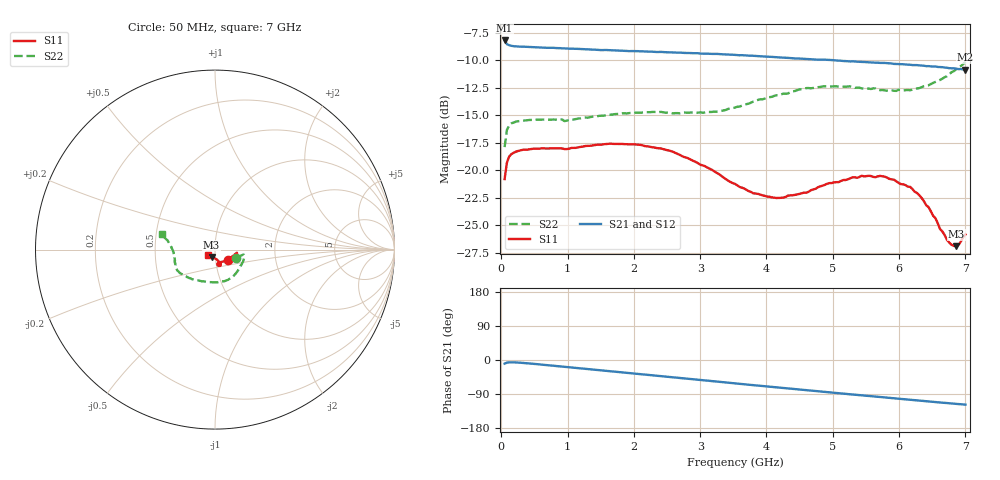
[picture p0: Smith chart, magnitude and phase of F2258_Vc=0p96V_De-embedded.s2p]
! Integrated Device Technology
! Corporate Headquarters
! 6024 Silver Creek Valley Road
! San Jose, CA 95138  USA
! Phone:  1-408-284-8200
! Toll Free:  1-800-223-1366
! Webpage:  http://www.idt.com/
! Timing and RF Division
! 515 Groton Road, Suite 102
! Westford, MA 01886-6024
! Device:  F2258
! Description: Voltage Variable RF Attenuator
! Frequency:  50.0 -  6000.00 MHz
! Package:  3x3 mm Thin QFN Plastic Package: 16 pin
! Ports:  2 RF, 2 DC
!  Pin  1  = NC
!  Pin  2  = NC
!  Pin  3  = RF2  = Port 2
!  Pin  4  = GND
!  Pin  5  = Vdd
!  Pin  6  = NC
!  Pin  7  = VCTRL
!  Pin  8  = NC
!  Pin  9  = GND
!  Pin 10  = RF1  = Port 1
!  Pin 11  = NC
!  Pin 12  = NC
!  Pin 13  = NC
!  Pin 14  = NC
!  Pin 15  = NC
!  Pin 16  = NC
! Vcntrl:  0.960 Volts
! Vdd:  +3.300 Volts
! Current:  1.153 mA
! Data:  The device was measured on a the F2258 evaluation board which has
!  individual transmission lines to the RF pins.  Data was collected
!  using a calibrated network analyzer.  The evaluation board was
!  de-embedded using a TRL calibration technique.
!  The reference plane is the edge of the package pin.
! Misc:  SN 10
!  Action Tracker AT0285
! Date Measured:  2014-12-10
! Date:  2016-01-13  MJV
! Note:
!  Integrated Device Technology supplies this data as a sample of measured
!  data at the package pin for this product.  Your particular data for this
!  product may vary.
!  Data was taken at 25 degrees C.
!  Integrated Device Technology reserves the right to change this data at anytime.
!Freq_(GHz)  S11M_(dB)  S11P_(deg)  S21M_(dB)  S21P_(deg)  S12M_(dB)  S12P_(deg)  S22M_(dB)  S22P_(deg)
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# GHz S dB R 50
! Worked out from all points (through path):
!   201 points, 50 MHz to 7 GHz, reference 50 ohm
!   highest |S21| = -8.21 dB at 50 MHz (marker M1); lowest = -10.9 dB at 7 GHz (marker M2)
!   group delay of S21, straight-line fit = 46.2 ps
!   lowest |S11| = -26.9 dB at 6.861 GHz (marker M3), VSWR 1.09, Z = 47.9 - j3.91 ohm
!   |S11| at or under -10 dB: start of sweep to end of sweep
!   |S22| runs from -17.9 to -10.2 dB; largest |S21 - S12| = 0.0019
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0.05  -20.82 -37.6  -8.21 -9.6  -8.19 -9.5  -17.91 -21.6
0.08475  -19.32 -18.1  -8.55 -7.0  -8.52 -7.0  -16.36 -11.9
0.1195  -18.76 -12.4  -8.65 -6.2  -8.63 -6.2  -15.92 -10.1
0.22375  -18.32 -8.6  -8.75 -6.4  -8.74 -6.4  -15.59 -10.6
0.9535  -18.09 -17.6  -8.94 -18.0  -8.91 -18.0  -15.55 -33.0
1.2315  -17.86 -20.2  -9.00 -22.7  -8.99 -22.7  -15.25 -41.5
1.6485  -17.60 -23.5  -9.09 -29.7  -9.09 -29.7  -14.96 -53.1
2.37825  -18.02 -27.6  -9.26 -41.9  -9.25 -41.9  -14.72 -73.0
2.83  -18.96 -31.9  -9.36 -49.6  -9.34 -49.6  -14.78 -87.8
3.525  -21.26 -47.9  -9.52 -61.7  -9.52 -61.7  -14.31 -114.9
3.803  -22.12 -59.0  -9.61 -66.5  -9.60 -66.5  -13.77 -125.4
4.1505  -22.54 -70.4  -9.74 -72.4  -9.73 -72.4  -13.20 -135.8
4.7065  -21.76 -80.5  -9.94 -81.6  -9.92 -81.6  -12.53 -148.4
5.43625  -20.51 -75.6  -10.16 -93.3  -10.16 -93.2  -12.57 -160.1
5.85325  -20.80 -70.0  -10.30 -99.9  -10.31 -99.9  -12.75 -168.6
6.166  -21.53 -68.6  -10.42 -104.9  -10.44 -104.8  -12.74 -176.0
6.305  -22.29 -69.8  -10.48 -107.1  -10.51 -107.1  -12.54 -179.7
6.54825  -24.37 -77.1  -10.58 -111.0  -10.60 -111.0  -11.98 174.0
6.61775  -25.36 -81.1  -10.63 -112.0  -10.65 -112.0  -11.80 172.1
6.722  -26.34 -92.3  -10.70 -113.7  -10.72 -113.7  -11.47 169.3
6.861  -26.92 -115.5  -10.78 -115.8  -10.79 -115.7  -10.84 166.8
7  -25.86 -141.0  -10.87 -117.8  -10.87 -117.9  -10.18 164.1
